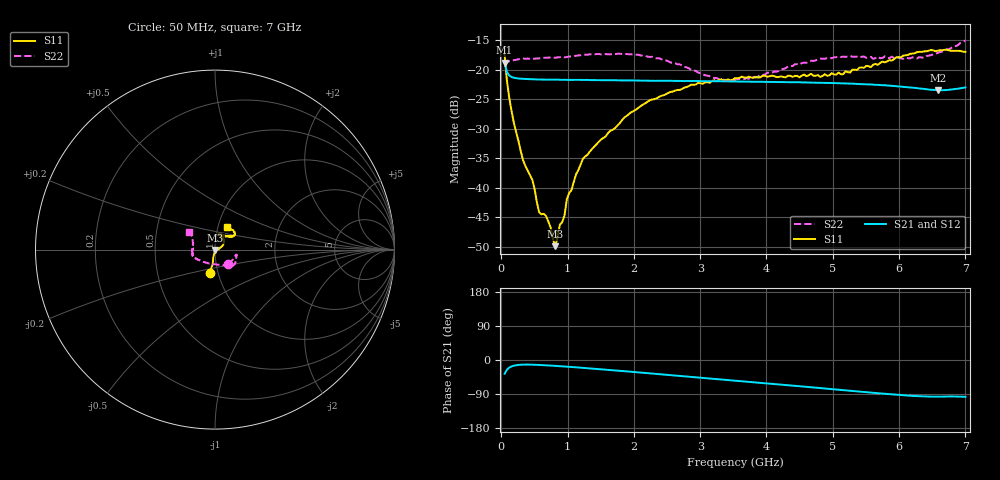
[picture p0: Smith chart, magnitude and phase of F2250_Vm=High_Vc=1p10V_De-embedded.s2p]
! Integrated Device Technology
! Corporate Headquarters
! 6024 Silver Creek Valley Road
! San Jose, CA 95138  USA
! Phone:  1-408-284-8200
! Toll Free:  1-800-223-1366
! Webpage:  http://www.idt.com/
! Timing and RF Division
! 515 Groton Road, Suite 102
! Westford, MA 01886-6024
! Device:  F2250
! Description: Voltage Variable RF Attenuator
! Frequency:  50.0 -  6000.00 MHz
! Package:  3x3 mm Thin QFN Plastic Package: 16 pin
! Ports:  2 RF, 3 DC
!  Pin  1  = GND
!  Pin  2  = NC
!  Pin  3  = RF1  = Port 1
!  Pin  4  = NC
!  Pin  5  = GND
!  Pin  6  = GND
!  Pin  7  = GND
!  Pin  8  = GND
!  Pin  9  = NC
!  Pin 10  = RF2  = Port 2
!  Pin 11  = NC
!  Pin 12  = GND
!  Pin 13  = GND
!  Pin 14  = VCNTRL
!  Pin 15  = VDD
!  Pin 16  = VMODE
! Vcntrl:  1.100 Volts
! Vmode:  +3.300 Volts
! Vdd:  +3.30  Volts
! Current:  1.328 mA
! Data:  The device was measured on a the F2250 evaluation board which has
!  individual transmission lines to the RF pins.  Data was collected
!  using a calibrated network analyzer.  The evaluation board was
!  de-embedded using a TRL calibration technique.
!  The reference plane is the edge of the package pin.
! Misc:  SN 10
!  Action Tracker AT0258
! Date Measured:  2014-11-26
! Date:  2015-10-15  MJV
! Note:
!  Integrated Device Technology supplies this data as a sample of measured
!  data at the package pin for this product.  Your particular data for this
!  product may vary.
!  Data was taken at 25 degrees C.
!  Integrated Device Technology reserves the right to change this data at anytime.
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# GHz S dB R 50
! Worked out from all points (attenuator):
!   201 points, 50 MHz to 7 GHz, reference 50 ohm
!   highest |S21| = -18.79 dB at 50 MHz (marker M1); lowest = -23.5 dB at 6.583 GHz (marker M2)
!   lowest |S11| = -49.9 dB at 814.5 MHz (marker M3), VSWR 1.01, Z = 50.3 - j0.169 ohm
!   |S11| at or under -10 dB: start of sweep to end of sweep
!   |S22| runs from -21.8 to -15.0 dB; largest |S21 - S12| = 0.00032
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0.05  -17.47 -103.0  -18.79 -36.4  -18.79 -36.4  -19.25 -47.8
0.08475  -21.84 -99.0  -20.40 -25.7  -20.42 -25.7  -18.65 -24.9
0.15425  -26.97 -102.4  -21.22 -16.9  -21.22 -16.9  -18.53 -15.0
0.328  -35.33 -100.7  -21.53 -12.2  -21.56 -12.2  -18.09 -13.0
0.467  -38.63 -102.0  -21.60 -12.3  -21.60 -12.3  -18.16 -14.7
0.57125  -44.16 -88.7  -21.65 -13.0  -21.66 -13.0  -18.09 -17.2
0.6755  -44.78 -78.4  -21.69 -14.0  -21.67 -14.0  -17.98 -19.1
0.745  -46.74 -61.5  -21.67 -14.7  -21.67 -14.7  -17.93 -20.7
0.8145  -49.88 -31.6  -21.68 -15.5  -21.69 -15.5  -17.96 -22.6
0.884  -46.23 -20.8  -21.70 -16.3  -21.70 -16.3  -17.87 -24.7
0.9535  -44.67 -29.2  -21.70 -17.1  -21.72 -17.2  -17.90 -25.8
0.98825  -41.97 -21.6  -21.72 -17.6  -21.72 -17.6  -17.85 -26.5
1.2315  -35.09 3.8  -21.73 -20.7  -21.73 -20.7  -17.45 -31.1
1.857  -28.08 23.1  -21.82 -29.6  -21.82 -29.6  -17.32 -39.7
2.37825  -24.61 35.5  -21.86 -37.1  -21.86 -37.1  -18.04 -47.4
3.1775  -21.90 56.6  -21.95 -49.0  -21.94 -49.1  -21.33 -76.6
3.525  -21.43 66.4  -22.00 -54.3  -22.01 -54.3  -21.70 -101.1
4.7065  -21.02 69.4  -22.19 -72.4  -22.19 -72.4  -18.50 -155.3
5.15825  -20.74 53.1  -22.31 -79.5  -22.32 -79.6  -17.77 -163.9
5.85325  -18.38 37.8  -22.69 -90.2  -22.69 -90.3  -18.03 -178.5
6.583  -16.77 43.0  -23.49 -96.7  -23.47 -96.9  -17.14 154.1
7  -16.97 61.9  -22.98 -97.2  -22.99 -97.2  -15.04 145.6
